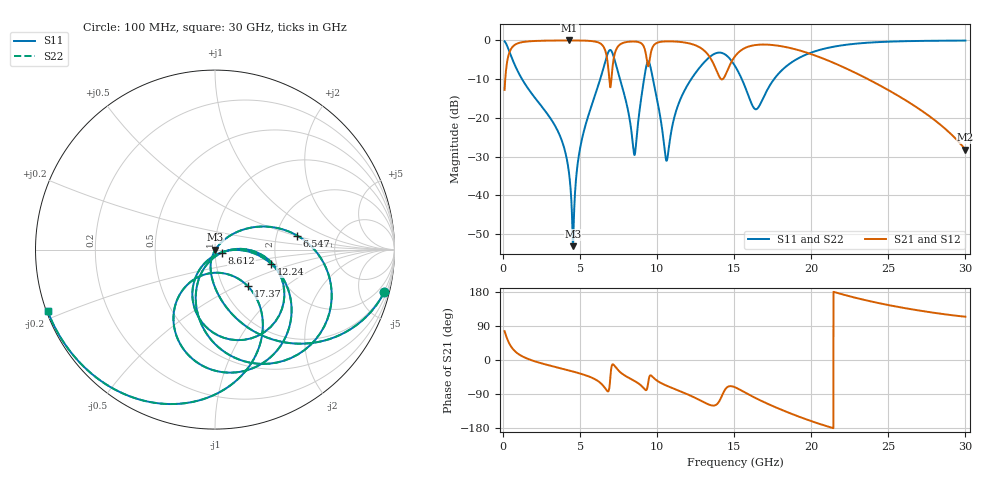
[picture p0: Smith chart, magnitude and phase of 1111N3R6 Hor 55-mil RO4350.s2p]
# GHz S MA R 50
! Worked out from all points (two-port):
!   3201 points, 100 MHz to 30 GHz, reference 50 ohm
!   highest |S21| = -0.02 dB at 4.305 GHz (marker M1); lowest = -28.2 dB at 30 GHz (marker M2)
!   |S21| within 3 dB of the highest: 420.8 MHz to 6.66 GHz (6.239 GHz wide, 176 % of centre); 15.3 GHz to 19.59 GHz (4.291 GHz wide, 24.6 % of centre)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
!   lowest |S11| = -53.1 dB at 4.538 GHz (marker M3), VSWR 1.00, Z = 50.2 - j0.117 ohm
!   |S11| at or under -10 dB: 1.231 GHz to 6.306 GHz (5.075 GHz wide, 135 % of centre); 9.728 GHz to 12.21 GHz (2.481 GHz wide, 22.6 % of centre); 15.49 GHz to 17.59 GHz (2.094 GHz wide, 12.7 % of centre)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
!   |S22| runs from -53.1 to -0.1 dB; largest |S21 - S12| = 0
!   S11 on the Smith chart (normalised r, x): 100 MHz: 0.91, -8.05; 6.547 GHz: 2.61, +0.52; 8.612 GHz: 1.08, -0.04; 12.24 GHz: 1.87, -0.33; 17.37 GHz: 1.30, -0.57; 30 GHz: 0.00, -0.18
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0.1  0.9731 -14.0  0.2301 76.0  0.2301 76.0  0.9731 -14.0
1.137156  0.3407 -77.7  0.9394 12.2  0.9394 12.2  0.3407 -77.7
3.557187  0.06715 -109.0  0.996 -20.1  0.996 -20.1  0.06715 -109.0
4.304688  0.01764 -111.7  0.9975 -27.9  0.9975 -27.9  0.01764 -111.7
4.538281  0.002206 -31.8  0.9973 -30.4  0.9973 -30.4  0.002206 -31.8
5.089563  0.04997 49.0  0.9946 -36.8  0.9946 -36.8  0.04997 49.0
6.547187  0.4642 9.7  0.8091 -70.5  0.8091 -70.5  0.4642 9.7
6.836844  0.7111 -24.2  0.4192 -82.1  0.4192 -82.1  0.7111 -24.2
7.107812  0.6766 -69.9  0.4617 -11.5  0.4617 -11.5  0.6766 -69.9
7.537625  0.3423 -107.5  0.8684 -29.8  0.8684 -29.8  0.3423 -107.5
8.612156  0.04229 -23.8  0.9635 -57.2  0.9635 -57.2  0.04229 -23.8
9.369  0.5232 -49.9  0.4937 -71.5  0.4937 -71.5  0.5232 -49.9
10.06978  0.1438 -127.5  0.9424 -56.7  0.9424 -56.7  0.1438 -127.5
10.63041  0.02829 -55.5  0.9712 -68.1  0.9712 -68.1  0.02829 -55.5
12.23753  0.3224 -14.2  0.8975 -95.5  0.8975 -95.5  0.3224 -14.2
14.05956  0.6954 -77.6  0.3315 -106.6  0.3315 -106.6  0.6954 -77.6
15.05  0.4669 -119.6  0.6224 -71.9  0.6224 -71.9  0.4669 -119.6
16.34878  0.1298 -94.0  0.869 -99.7  0.869 -99.7  0.1298 -94.0
17.36725  0.2734 -48.1  0.8754 -119.2  0.8754 -119.2  0.2734 -48.1
20.03956  0.7005 -76.2  0.6596 -161.8  0.6596 -161.8  0.7005 -76.2
25.01978  0.9625 -127.4  0.2269 144.8  0.2269 144.8  0.9625 -127.4
30  0.9936 -159.7  0.03883 114.2  0.03883 114.2  0.9936 -159.7
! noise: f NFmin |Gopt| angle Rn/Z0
0.1  0.001272  0.866  3.487  0.002038
3.417  0.009345  0.4622  24.43  0.002812
6.743  0.2013  0.9365  44.32  0.6069
10.06  0.09251  0.8128  64.63  0.074
13.39  0.2641  0.9106  82.99  0.3654
16.7  0.1826  0.8468  100.7  0.1043
20.03  0.1604  0.8016  115.9  0.04874
23.35  0.2121  0.833  130.2  0.04934
26.67  0.3701  0.8987  145.2  0.07357
30  1.111  0.9658  160.8  0.2097
